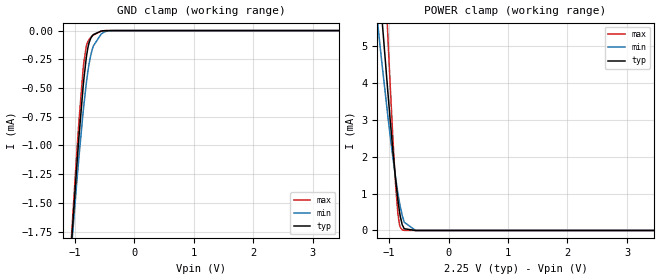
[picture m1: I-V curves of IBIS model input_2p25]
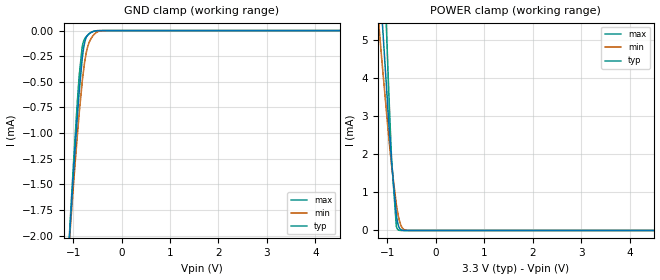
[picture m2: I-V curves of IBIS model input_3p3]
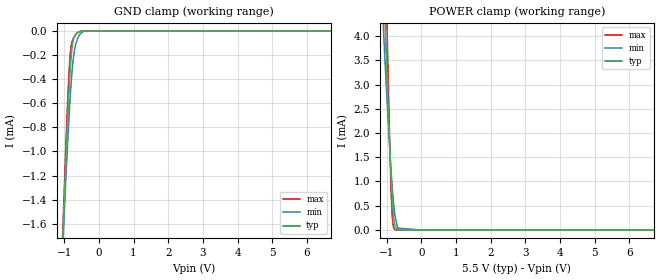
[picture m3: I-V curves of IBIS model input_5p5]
| Texas Instruments Incorporated
| SN74HCS595 8-bit shift register with Schmitt-trigger inputs
| and 3-state output registers
[IBIS Ver]   4.1
[File name]   sn74hcs595.ibs
[File Rev]   1.0
[Date]   02/26/2021
[Source]
| Texas Instruments Incorporated.
| Analog-eLab Design Center, HPA
| 12500 TI Blvd
| Dallas, TX -75243
[Notes]   Revision History:
| Rev 1.0: 02/26/2021
| - Initial version of the model
| - Model generated from simulations in SPECTRE
| - C_comp although listed in numerical order of value are
|   obtained from varying PVT conditions. For PVT conditions for
|   each specific value refer the buffer description under
|   respective [Model]. IBIS model user is responsible for using
|   appropriate C_comp to simulate for Signal Integrity.
| - Warnings regarding combined Non-monotonicity of various models have been
|   reviewed and considered minor and can be ignored.
| - Model names with a trailing _2p25 contain the model for 2.25V operation.
|   Model names with a trailing _3p3 contain the model for 3.3V operation.
|   Model names with a trailing _5p5 contain the model for 5.5V operation.
[Disclaimer]
| This model is designed as an aid for customers of Texas Instruments.
| TI and its licensors and suppliers make no warranties, either expressed
| or implied, with respect to this  model, including the warranties of
| merchantability or fitness for a particular purpose. The model is
| provided solely on an "as is" basis. The entire risk as to its quality
| and performance is with the customer.
| This model is subject to change without notice. Texas Instruments
| Incorporated is not responsible for updating this model.
[Copyright]
 (C) Copyright 2021 Texas Instruments Incorporated. All rights reserved.
|  Component SN74HCS595DYY 16-Pin SOT-23 THIN - DYY package
|  Part # SN74HCS595DYYR
[Component]   SN74HCS595DYY
[Manufacturer]   TI
[Package]   |16 SOT-23 THIN - DYY package
|   typ   min   max
R_pkg   0.05   0.04   0.06
L_pkg   1.0nH   0.8nH   1.2nH
C_pkg   0.2pF   0.16pF   0.24pF
[Pin]   signal_name   model_name   R_pin   L_pin   C_pin
1   QB   output   NA   NA   NA
2   QC   output   NA   NA   NA
3   QD   output   NA   NA   NA
4   QE   output   NA   NA   NA
5   QF   output   NA   NA   NA
6   QG   output   NA   NA   NA
7   QH   output   NA   NA   NA
8   GND   gnd   NA   NA   NA
9   QH'   output   NA   NA   NA
10   SRCLR_NOT   input   NA   NA   NA
11   SRCLK   input   NA   NA   NA
12   RCLK   input   NA   NA   NA
13   OE_NOT   input   NA   NA   NA
14   SER   input   NA   NA   NA
15   QA   output   NA   NA   NA
16   VCC   power   NA   NA   NA
|  Component SN74HCS595D 16-Pin SOIC - D package
|  Part # SN74HCS595DR
[Component]   SN74HCS595D
[Manufacturer]   TI
[Package]   |16 SOIC - D package
|   typ   min   max
R_pkg   0.05   0.04   0.06
L_pkg   1.0nH   0.8nH   1.2nH
C_pkg   0.2pF   0.16pF   0.24pF
[Pin]   signal_name   model_name   R_pin   L_pin   C_pin
1   QB   output   NA   NA   NA
2   QC   output   NA   NA   NA
3   QD   output   NA   NA   NA
4   QE   output   NA   NA   NA
5   QF   output   NA   NA   NA
6   QG   output   NA   NA   NA
7   QH   output   NA   NA   NA
8   GND   gnd   NA   NA   NA
9   QH'   output   NA   NA   NA
10   SRCLR_NOT   input   NA   NA   NA
11   SRCLK   input   NA   NA   NA
12   RCLK   input   NA   NA   NA
13   OE_NOT   input   NA   NA   NA
14   SER   input   NA   NA   NA
15   QA   output   NA   NA   NA
16   VCC   power   NA   NA   NA
|  Component SN74HCS595BQB 16-Pin WQFN - BQB package
|  Part # SN74HCS595BQBR
[Component]   SN74HCS595BQB
[Manufacturer]   TI
[Package]   |16 WQFN - BQB package
|   typ   min   max
R_pkg   0.05   0.04   0.06
L_pkg   1.0nH   0.8nH   1.2nH
C_pkg   0.2pF   0.16pF   0.24pF
[Pin]   signal_name   model_name   R_pin   L_pin   C_pin
1   QB   output   NA   NA   NA
2   QC   output   NA   NA   NA
3   QD   output   NA   NA   NA
4   QE   output   NA   NA   NA
5   QF   output   NA   NA   NA
6   QG   output   NA   NA   NA
7   QH   output   NA   NA   NA
8   GND   gnd   NA   NA   NA
9   QH'   output   NA   NA   NA
10   SRCLR_NOT   input   NA   NA   NA
11   SRCLK   input   NA   NA   NA
12   RCLK   input   NA   NA   NA
13   OE_NOT   input   NA   NA   NA
14   SER   input   NA   NA   NA
15   QA   output   NA   NA   NA
16   VCC   power   NA   NA   NA
|  Component SN74HCS595PW 16-Pin TSSOP - PW package
|  Part # SN74HCS595PWR
[Component]   SN74HCS595PW
[Manufacturer]   TI
[Package]   |16 TSSOP - PW package
|   typ   min   max
R_pkg   0.05   0.04   0.06
L_pkg   1.0nH   0.8nH   1.2nH
C_pkg   0.2pF   0.16pF   0.24pF
[Pin]   signal_name   model_name   R_pin   L_pin   C_pin
1   QB   output   NA   NA   NA
2   QC   output   NA   NA   NA
3   QD   output   NA   NA   NA
4   QE   output   NA   NA   NA
5   QF   output   NA   NA   NA
6   QG   output   NA   NA   NA
7   QH   output   NA   NA   NA
8   GND   gnd   NA   NA   NA
9   QH'   output   NA   NA   NA
10   SRCLR_NOT   input   NA   NA   NA
11   SRCLK   input   NA   NA   NA
12   RCLK   input   NA   NA   NA
13   OE_NOT   input   NA   NA   NA
14   SER   input   NA   NA   NA
15   QA   output   NA   NA   NA
16   VCC   power   NA   NA   NA
|   Model Selectors
[Model Selector] input
input_2p25   2.25V   digital input
input_3p3   3.3V   digital input
input_5p5   5.5V   digital input
[Model Selector] output
output_2p25   2.25V   digital output
output_3p3   3.3V   digital output
output_5p5   5.5V   digital output
| Models and submodels in the file (6): input_2p25 (Input), input_3p3 (Input), input_5p5 (Input), output_2p25 (3-state), output_3p3 (3-state), output_5p5 (3-state)
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|   input_2p25 Model
[Model]   input_2p25
Model_type   Input
Vinl = 0.835
Vinh = 1.1
|   typ   min   max
C_comp   0.119pF   0.105pF   0.126pF
| Where Nom  PVT is Nominal Process, 2.25V, 27C
|   Fast PVT is Strong Process,  2.50V, -55C
|   Slow PVT is Weak Process,   2.0V, 150C
[Voltage Range]   2.25   2   2.5
|Junction Temperature
[Temperature Range]   27   150   -55
[Power Clamp Reference]   2.25   2   2.5
[GND Clamp Reference]   0   0   0
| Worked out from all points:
|   GND clamp passes 1 mA (typ) near -0.94 V on its own axis
|   POWER clamp passes 1 mA (typ) near -0.86 V on its own axis
[GND Clamp]
|   Voltage   I(typ)   I(min)   I(max)
-2.25V    -11.71mA   -10.48mA   -12.74mA
-1.109V   -2.268mA   -2.257mA   -2.25mA
-967.5mV  -1.202mA   -1.339mA   -1.088mA
-927mV    -920.7uA   -1.094mA   -783.1uA
-846mV    -425uA     -650.3uA   -278.1uA
-805.5mV  -239.4uA   -463.5uA   -138.6uA
-771.8mV  -134.7uA   -334.5uA   -88.4uA
-731.2mV  -67.91uA   -218.2uA   -59.95uA
-684mV    -34.91uA   -132.4uA   -37.48uA
-555.7mV  -4.734uA   -31.52uA   -3.97uA
-393.7mV  -80nA      -1.094uA   -16.84nA
4.5V      0A         0A         0A
[POWER Clamp]
|   Voltage   I(typ)   I(min)   I(max)
-2.25V    34.95mA    23.58mA    64.72mA
-1.386V   11.37mA    8.623mA    18.57mA
-1.143V   6.234mA    4.883mA    9.607mA
-1.123V   5.818mA    4.582mA    8.877mA
-1.015V   3.652mA    3.027mA    5.08mA
-940.5mV  2.258mA    2.037mA    2.657mA
-893.2mV  1.451mA    1.465mA    1.318mA
-852.8mV  850.3uA    1.028mA    472.1uA
-819mV    453.9uA    713.6uA    125uA
-778.5mV  153.7uA    408.4uA    17.82uA
-555.7mV  28.75nA    1.244uA    0A
4.5V      0A         0A         0A
|   input_3p3 Model
[Model]   input_3p3
Model_type   Input
Vinl = 1.6
Vinh = 2.3
|   typ   min   max
C_comp   0.1147pF   0.0972pF   0.1185pF
| Where Nom  PVT is Nominal Process, 3.3V, 27C
|   Fast PVT is Strong Process,  3.6V, -55C
|   Slow PVT is Weak Process,   3.0V, 150C
[Voltage Range]   3.3   3   3.6
|Junction Temperature
[Temperature Range]   27   150   -55
[Power Clamp Reference]   3.3   3   3.6
[GND Clamp Reference]   0   0   0
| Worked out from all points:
|   GND clamp passes 1 mA (typ) near -0.94 V on its own axis
|   POWER clamp passes 1 mA (typ) near -0.86 V on its own axis
[GND Clamp]
|   Voltage   I(typ)   I(min)   I(max)
-3.3V     -20.63mA   -18.3mA    -22.65mA
-1.132V   -2.445mA   -2.409mA   -2.444mA
-1.043V   -1.757mA   -1.817mA   -1.692mA
-963.6mV  -1.175mA   -1.315mA   -1.058mA
-894.3mV  -706.6uA   -906.4uA   -555.8uA
-874.5mV  -585.2uA   -797.8uA   -431.1uA
-815.1mV  -278uA     -505uA     -162.5uA
-775.5mV  -143.9uA   -347.5uA   -92.16uA
-726mV    -62.63uA   -206.2uA   -57.12uA
-607.2mV  -11.96uA   -59.92uA   -12.28uA
-379.5mV  -51.1nA    -764.7nA   -8.033nA
6.6V      0A         0A         0A
[POWER Clamp]
|   Voltage   I(typ)   I(min)   I(max)
-3.3V     78.77mA    53.53mA    141.7mA
-1.221V   7.859mA    6.061mA    12.45mA
-1.122V   5.802mA    4.57mA     8.85mA
-1.112V   5.6mA      4.424mA    8.495mA
-983.4mV  3.05mA     2.598mA    4.028mA
-914.1mV  1.796mA    1.71mA     1.877mA
-815.1mV  416uA      680.5uA    104.6uA
-765.6mV  100.2uA    329.9uA    9.392uA
-726mV    22.82uA    150.2uA    1.327uA
-686.4mV  4.733uA    56.24uA    192.9nA
-557.7mV  30.26nA    1.317uA    0A
6.6V      0A         0A         0A
|   input_5p5 Model
[Model]   input_5p5
Model_type   Input
Vinl = 2.45
Vinh = 3.0
|   typ   min   max
C_comp   0.107pF   0.087pF   0.107pF
| Where Nom  PVT is Nominal Process, 5.5V, 27C
|   Fast PVT is Strong Process,  6.0V, -55C
|   Slow PVT is Weak Process,   5.0V, 150C
[Voltage Range]   5.5   5   6
|Junction Temperature
[Temperature Range]   27   150   -55
[Power Clamp Reference]   5.5   5   6
[GND Clamp Reference]   0   0   0
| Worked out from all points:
|   GND clamp passes 1 mA (typ) near -0.94 V on its own axis
|   POWER clamp passes 1 mA (typ) near -0.86 V on its own axis
[GND Clamp]
|   Voltage   I(typ)   I(min)   I(max)
-2.5V     -13.83mA   -12.33mA   -15.1mA
-1.04V    -1.74mA    -1.802mA   -1.673mA
-1.03V    -1.661mA   -1.734mA   -1.587mA
-1.009V   -1.504mA   -1.599mA   -1.416mA
-904mV    -768.6uA   -961.1uA   -620.9uA
-830.5mV  -347.2uA   -575.3uA   -212.7uA
-778mV    -150.4uA   -356.3uA   -94.85uA
-715mV    -53.22uA   -183.3uA   -51.53uA
-578.5mV  -7.325uA   -42.74uA   -6.817uA
-431.5mV  -235nA     -2.752uA   -78nA
-22mV     0A         0A         0A
8V        0A         0A         0A
[POWER Clamp]
|   Voltage   I(typ)   I(min)   I(max)
-2.5V     44.53mA    30.06mA    82.85mA
-1.093V   5.211mA    4.144mA    7.813mA
-1.051V   4.366mA    3.537mA    6.331mA
-1.02V    3.745mA    3.093mA    5.242mA
-956.5mV  2.548mA    2.242mA    3.156mA
-893.5mV  1.455mA    1.468mA    1.324mA
-851.5mV  833.6uA    1.016mA    453uA
-820mV    463.9uA    722.1uA    130.7uA
-757mV    73.97uA    282.9uA    6.127uA
-673mV    2.776uA    39uA       100.5nA
-22mV     0A         0A         0A
8V        0A         0A         0A
